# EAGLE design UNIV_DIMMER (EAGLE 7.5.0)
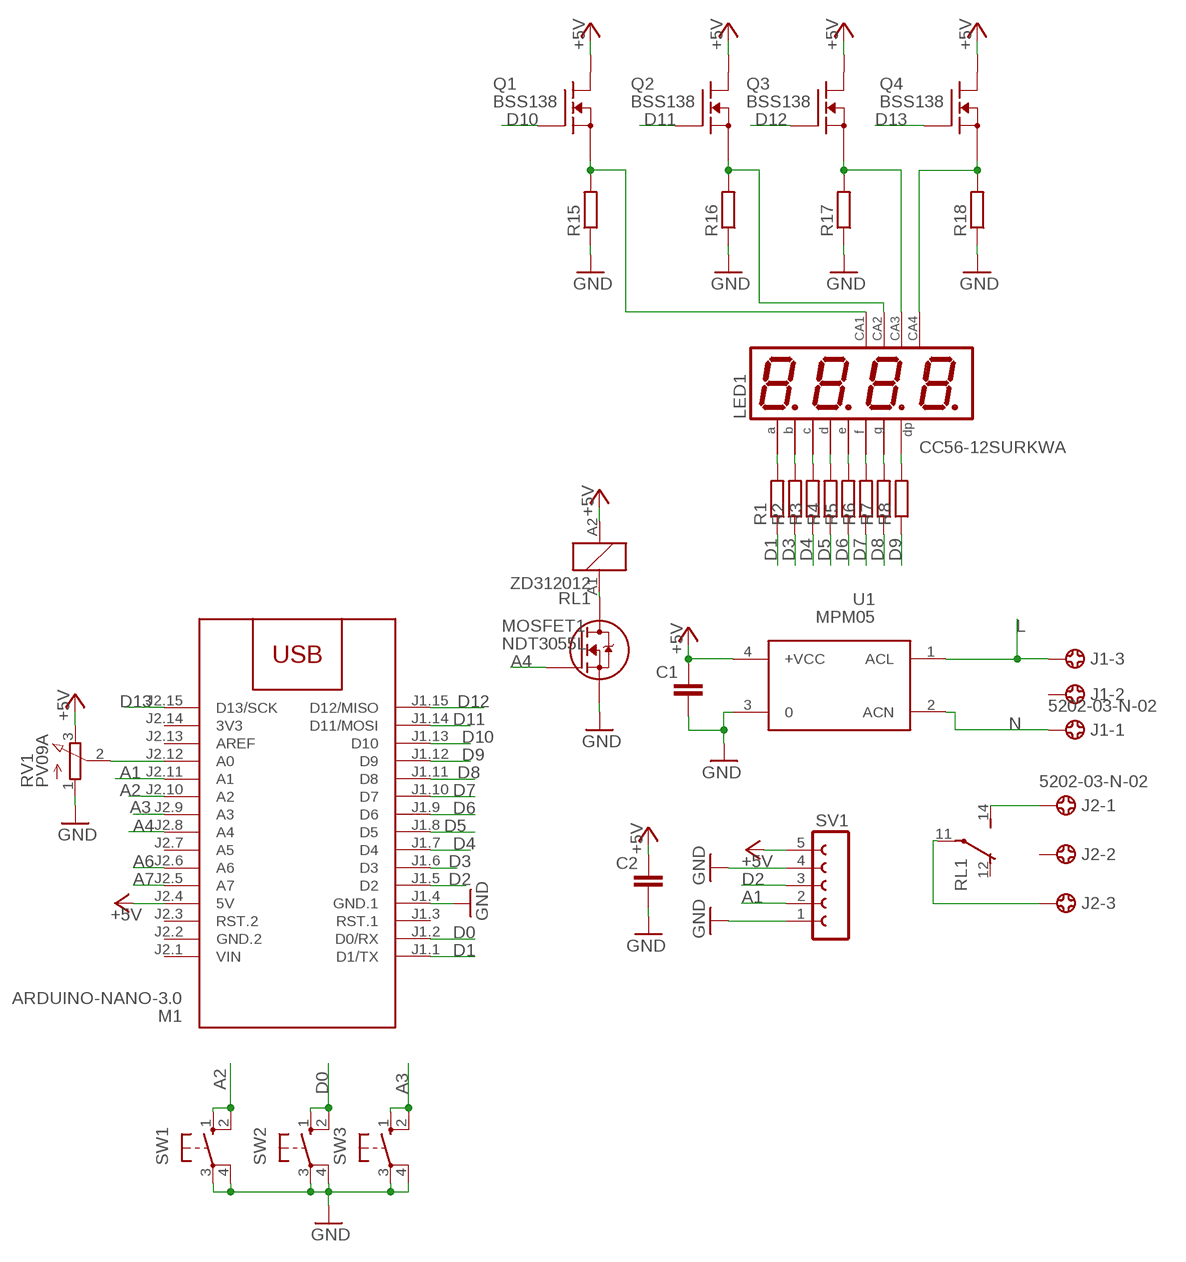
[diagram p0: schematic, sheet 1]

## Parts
C1  C-EUC1206  [C1206]
C2  C-EUC1206  [C1206]
J1  5202-03-N-02  [5202-03-N-02]
J2  5202-03-N-02  [5202-03-N-02]
LED1  CC56-12SURKWA  CA56-12SURKWA  [CA56-12SURKWA]
M1  ARDUINO-NANO-3.0  [ARDUINO-NANO-3.0]
MOSFET1  NDT3055L  [SOT223-4]
Q1  BSS138  [SOT23]
Q2  BSS138  [SOT23]
Q3  BSS138  [SOT23]
Q4  BSS138  [SOT23]
R1  R-EU_R1206  [R1206]
R2  R-EU_R1206  [R1206]
R3  R-EU_R1206  [R1206]
R4  R-EU_R1206  [R1206]
R5  R-EU_R1206  [R1206]
R6  R-EU_R1206  [R1206]
R7  R-EU_R1206  [R1206]
R8  R-EU_R1206  [R1206]
R15  R-EU_R1206  [R1206]
R16  R-EU_R1206  [R1206]
R17  R-EU_R1206  [R1206]
R18  R-EU_R1206  [R1206]
RL1  ZD312012  [ZD1]
RV1  PV09A  [PTV09]
SV1  FE05-1  [FE05-1]
SW1  10-XX  [B3F-10XX]
SW2  10-XX  [B3F-10XX]
SW3  10-XX  [B3F-10XX]
U1  MPM05  [MPM05]

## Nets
+5V: C1.1 C2.1 M1.J2.4(5V) Q1.2(D) Q2.2(D) Q3.2(D) Q4.2(D) RL1.A2 RV1.3(E) SV1.5 U1.4(+VCC)
A1: M1.J2.11(A1) SV1.2
A2: M1.J2.10(A2) SW1.1(S) SW1.2(S1)
A3: M1.J2.9(A3) SW3.1(S) SW3.2(S1)
A4: M1.J2.8(A4) MOSFET1.1(G)
A6: M1.J2.6(A6)
A7: M1.J2.5(A7)
D0: M1.J1.2(D0/RX) SW2.1(S) SW2.2(S1)
D1: M1.J1.1(D1/TX) R1.1
D2: M1.J1.5(D2) SV1.3
D3: M1.J1.6(D3) R2.1
D4: M1.J1.7(D4) R3.1
D5: M1.J1.8(D5) R4.1
D6: M1.J1.9(D6) R5.1
D7: M1.J1.10(D7) R6.1
D8: M1.J1.11(D8) R7.1
D9: M1.J1.12(D9) R8.1
D10: M1.J1.13(D10) Q1.3(G)
D11: M1.J1.14(D11/MOSI) Q2.3(G)
D12: M1.J1.15(D12/MISO) Q3.3(G)
D13: M1.J2.15(D13/SCK) Q4.3(G)
GND: C1.2 C2.2 M1.J1.4(GND.1) MOSFET1.3(S) R15.1 R16.1 R17.1 R18.1 RV1.1(A) SV1.1 SV1.4 SW1.3(P) SW1.4(P1) SW2.3(P) SW2.4(P1) SW3.3(P) SW3.4(P1) U1.3
L: J1.3 U1.1(ACL)
N: J1.1 U1.2(ACN)
N$1: M1.J2.12(A0) RV1.2(S)
N$2: J2.1 RL1.14(2:S)
N$3: J2.3 RL1.11(2:P)
N$10: LED1.11(A) R1.2
N$11: LED1.7(B) R2.2
N$12: MOSFET1.2(D) MOSFET1.4(D) RL1.A1
N$15: LED1.4(C) R3.2
N$16: LED1.2(D) R4.2
N$17: LED1.1(E) R5.2
N$18: LED1.10(F) R6.2
N$19: LED1.5(G) R7.2
N$20: LED1.3(DP) R8.2
N$21: LED1.12(CA) Q1.1(S) R15.2
N$22: LED1.9(CA) Q2.1(S) R16.2
N$23: LED1.8(CA) Q3.1(S) R17.2
N$24: LED1.6(CA4) Q4.1(S) R18.2
Unconnected: J1.2 J2.2 M1.J1.3(RST.1) M1.J2.3(RST.2) M1.J2.7(A5) M1.J2.13(AREF) RL1.12(2:O)

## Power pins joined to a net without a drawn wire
3V3: M1.J2.14(3V3)
GND.2: M1.J2.2(GND.2)
VIN: M1.J2.1(VIN)

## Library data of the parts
C1 C2 = rcl:C-EU: CAPACITOR, European symbol
J1 J2 = con-ebyelectro:5202-03-N-02: Barrier Blocks Sreies 5202 Source: http://www.ebyelectro.com/PDF/5202-XX-N-02.pdf; OC_FARNELL: unknown; OC_NEWARK: unknown
LED1 = display-kingbright:CA56-12SURKWA
M1 = diy-modules:ARDUINO-NANO-3.0: Arduino Nano 3.0 and compatible devices More details available here: https://www.arduino.cc/en/Main/ArduinoBoardNano Click here to find device on ebay.com
MOSFET1 = NDT3055L:NDT3055L: Trans MOSFET N-CH 60V 4A 4-Pin(3+Tab) SOT-223 Trans MOSFET N-CH 60V 4A 4-Pin(3+Tab) SOT-223 Check availability; AVAILABILITY: In Stock; CHECK_PRICES: https://www.snapeda.com/parts/NDT3055L/Onsemi/view-part/?ref=eda; DESCRIPTION: Trans MOSFET N-CH 60V 4A 4-Pin(3+Tab) SOT-223 Trans MOSFET N-CH 60V 4A 4-Pin(3+Tab) SOT-223; MF: ON; MP: NDT3055L; PACKAGE: SOT-223-4 Fairchild Semiconductor; PRICE: None; SNAPEDA_LINK: https://www.snapeda.com/parts/NDT3055L/Onsemi/view-part/?ref=snap
Q1-Q4 = transistor-fet:BSS138
R1-R8 R15-R18 = rcl:R-EU_: RESISTOR, European symbol
RL1 = relay:ZD?1*: Power Relay SCHRACK 1 pole 30 A Source: http://www.schrack.com/.. 5848.pdf; OC_FARNELL: unknown; OC_NEWARK: unknown
RV1 = pot:PV09A
SV1 = con-lsta:FE05-1: FEMALE HEADER; OC_FARNELL: unknown; OC_NEWARK: unknown
SW1-SW3 = switch-omron:10-XX: OMRON SWITCH; MPN: B3F-1000; OC_FARNELL: 176432; OC_NEWARK: 36M3542
U1 = acdc:MPM05: AC DC Converter 5W

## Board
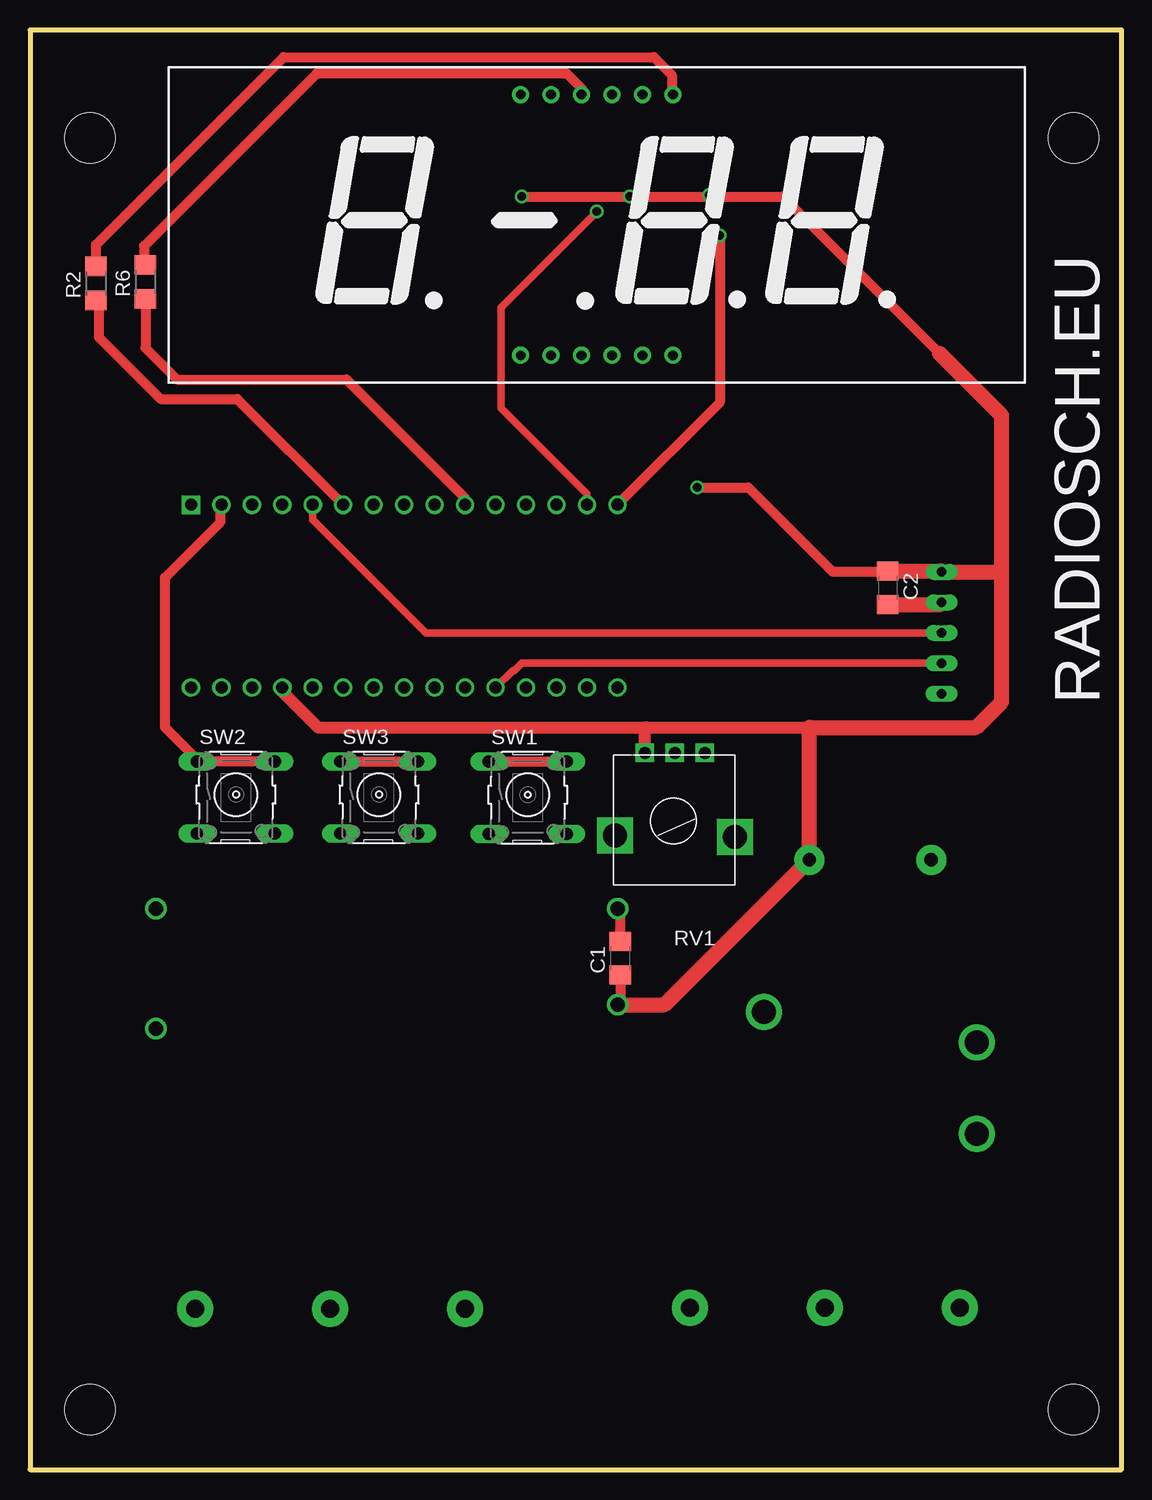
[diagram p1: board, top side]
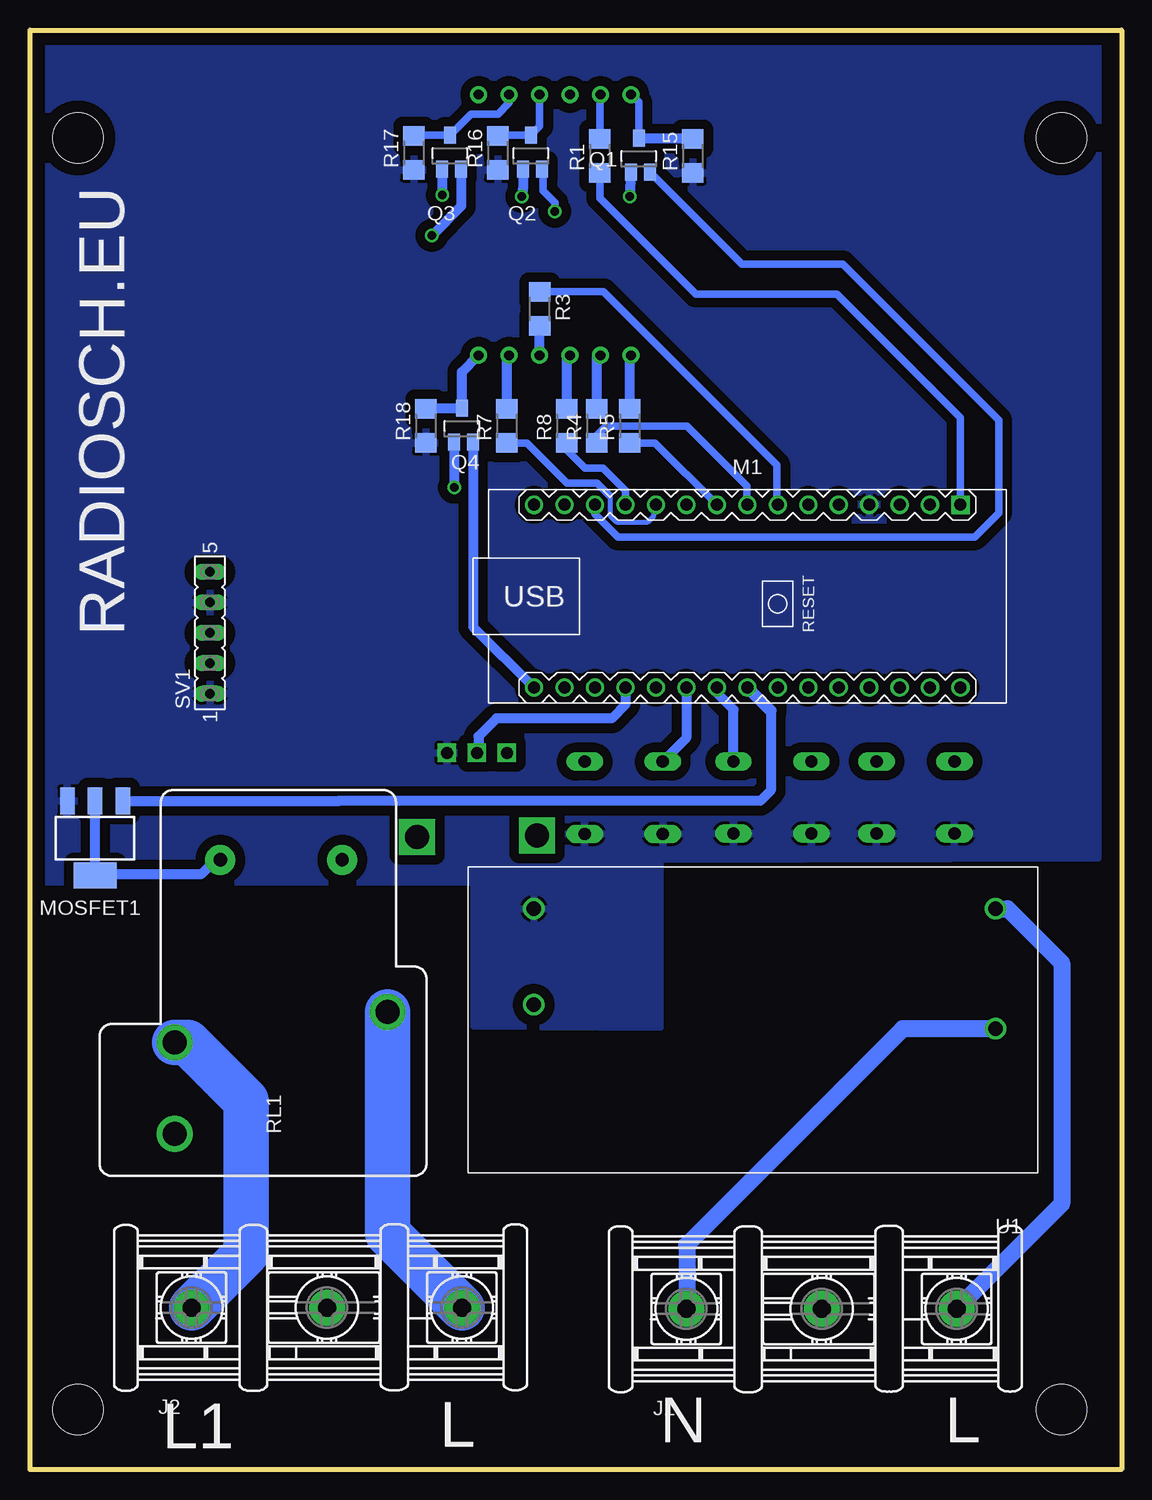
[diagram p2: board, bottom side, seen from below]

Size 91 x 120 mm. Coordinates in mm from the lower left corner, seen from the top.
Outline: 0,0 91,0 91,120 0,120 0,0
Copper layers (1*16): Top 0.035mm / dielectric 1.5mm / Bottom 0.035mm
Design rules "default": minimum track width 10mil, minimum drill 24mil, track to track 8mil, track to pad 8mil, pad to pad 8mil, via to via 8mil, smd to smd 8mil, copper to edge 40mil, drill to drill 8mil, minimum pad ring 10mil, minimum via ring 8mil, stop-mask expansion 4mil, vias tented up to drill 0mil, thermal gap 10mil
Holes 4.2 mm at 5,111 5,5 87,111 87,5

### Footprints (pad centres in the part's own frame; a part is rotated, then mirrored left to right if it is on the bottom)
C1206 = smd 1.6 x 1.8: 1 -1.4,0; 2 1.4,0
5202-03-N-02 = drill 1.5 pad 3: 1 -9.29,0; 2 2,0; 3 13.25,0
CA56-12SURKWA = drill 0.8 pad 1.422: 1 10.65,-7.12; 2 13.19,-7.12; 3 15.73,-7.12; 4 18.27,-7.12; 5 20.81,-7.12; 6 23.35,-7.12; 7 23.35,14.62; 8 20.81,14.62; 9 18.27,14.62; 10 15.73,14.62; 11 13.19,14.62; 12 10.65,14.62
ARDUINO-NANO-3.0 = drill 1 square: J1.1 17.78,7.62 | drill 1: J1.2 15.24,7.62; J1.3 12.7,7.62; J1.4 10.16,7.62; J1.5 7.62,7.62; J1.6 5.08,7.62; J1.7 2.54,7.62; J1.8 0,7.62; J1.9 -2.54,7.62; J1.10 -5.08,7.62; J1.11 -7.62,7.62; J1.12 -10.16,7.62; J1.13 -12.7,7.62; J1.14 -15.24,7.62; J1.15 -17.78,7.62; J2.1 17.78,-7.62; J2.2 15.24,-7.62; J2.3 12.7,-7.62; J2.4 10.16,-7.62; J2.5 7.62,-7.62; J2.6 5.08,-7.62; J2.7 2.54,-7.62; J2.8 0,-7.62; J2.9 -2.54,-7.62; J2.10 -5.08,-7.62; J2.11 -7.62,-7.62; J2.12 -10.16,-7.62; J2.13 -12.7,-7.62; J2.14 -15.24,-7.62; J2.15 -17.78,-7.62
SOT223-4 = smd 1.219 x 2.235: 1 -2.24,-3.091; 2 0.071,-3.091; 3 2.383,-3.091 | smd 3.6 x 2.2: 4 0.071,3.107
SOT23 = smd 1 x 1.4: 1 0,1.735; 2 -0.632,-1.1; 3 0.95,-1.1
R1206 = smd 1.6 x 1.803: 1 -1.422,0; 2 1.422,0
ZD1 = drill 2 pad 2.5: 11 -2.54,-8.88; 12 -12.7,8.88; 14 -5.08,8.88 | drill 1.1 pad 2.5: A1 10.16,5.08; A2 10.16,-5.08
PTV09 = drill 1 square: 1 -2.5,0; 2 0,0; 3 2.5,0 | drill 2 square: P$4 -5,7; P$5 5,6.9
FE05-1 = drill 0.813 long: 1 -5.08,0; 2 -2.54,0; 3 0,0; 4 2.54,0; 5 5.08,0
B3F-10XX = drill 1.016 long: 1 -3.251,2.761; 2 3.251,2.761; 3 -3.251,-3.261; 4 3.251,-3.261
MPM05 = drill 1.2: 1 3.5,-22; 2 3.5,-12; 3 42,-22; 4 42,-14

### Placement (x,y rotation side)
C1  49.22,42.62 90 top
C2  71.5,73.5 270 top
J1  27,13.39 0 bottom
J2  68.25,13.5 0 bottom
LED1  30.25,100 0 top
M1  31.2,72.8 0 bottom
MOSFET1  85.5,52.62 180 bottom
Q1  40.25,109.25 0 bottom
Q2  49.25,109.5 0 bottom
Q3  56,109.5 0 bottom
Q4  55,86.75 0 bottom
R1  43.5,109.5 90 bottom
R2  5.5,98.88 90 top
R3  48.5,96.75 270 bottom
R4  43.75,87 90 bottom
R5  41,87 90 bottom
R6  9.62,99 90 top
R7  51.25,87 90 bottom
R8  46.25,87 90 bottom
R15  35.75,109.5 90 bottom
R16  52,109.75 90 bottom
R17  59,109.75 90 bottom
R18  58,87 90 bottom
RL1  70.05,40.67 90 bottom
RV1  53.75,59.75 180 top
SV1  76,69.75 90 bottom
SW1  41.5,56.25 0 top
SW2  17.17,56.27 0 top
SW3  29.1,56.27 0 top
U1  7,24.75 180 bottom

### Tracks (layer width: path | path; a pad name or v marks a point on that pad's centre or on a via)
+5V  (via drill 0.7)
  Top 0.813: v41,106.12 v50,106.12 56.5,106.12 | 56.5,106.12 v56.62,106.25 | 56.5,106.12 62.75,106.12 75.81,93.06 76,92.88 | v55.62,81.88 59.88,81.88 66.88,74.88 71.47,74.88 C2.1 | C1.1 49.22,38.97 U1.4
  Top 1.016: M1.J2.4 21.04,64.84 24,61.88 51.38,61.88 | 51.38,61.88 65,61.88 | RV1.3 51.25,61.75 51.38,61.88
  Top 1.27: U1.4 52.89,38.75 RL1.A2 64.97,61.84 65,61.88 78.88,61.88 81,64 81,74.75 | 81,74.75 81,87.88 75.81,93.06 | 81,74.75 80.92,74.83 SV1.5 75.93,74.9 C2.1
  Bottom 0.61: 55.5,81.75 v55.62,81.88
  Bottom 0.813: v41,106.12 Q1.2 | Q2.2 49.88,107.01 v50,106.12 | Q3.2 56.63,107.12 v56.62,106.25 | Q4.2 55.63,81.88 v55.62,81.88
A1
  Top 0.61: M1.J2.11 40.27,66.62 40.38,66.62 41,67.25 75.96,67.25 SV1.2
A2
  Top 0.813: SW1.1 SW1.2
  Bottom 0.813: M1.J2.10 36.28,60.98 SW1.1
A3
  Top 0.813: SW3.1 SW3.2
  Bottom 0.813: SW3.2 32.35,63.35 33.62,64.62 33.62,65.06 M1.J2.9
A4
  Bottom 0.813: 29.25,63.23 29.25,56.62 30.12,55.75 65.25,55.75 65.28,55.72 MOSFET1.1
  Bottom 1.016: 29.25,63.23 M1.J2.8
D0
  Top 0.813: M1.J1.2 15.88,80.33 15.88,79 11.25,74.38 11.25,61.88 13.92,59.21 SW2.1 SW2.2
D1
  Bottom 0.61: M1.J1.1 13.42,87.67 23.75,98 35.5,98 43.5,106 R1.1
D2
  Top 0.61: M1.J1.5 23.58,79.17 33,69.75 SV1.3
D3
  Top 0.813: R2.1 5.75,97.2 5.75,94.38 10.88,89.25 17.29,89.25 M1.J1.6
D4
  Bottom 0.61: R3.1 43.17,98.17 28.75,83.75 28.75,80.51 M1.J1.7
D5
  Bottom 0.61: M1.J1.8 31.25,80.47 31.25,82 36.25,87 43,87 43.75,86.25 R4.1
D6
  Bottom 0.61: R5.1 38.9,85.58 M1.J1.9
D7
  Top 0.813: R6.1 9.62,93.5 12.25,90.88 26.38,90.88 36.25,81 36.25,80.45 M1.J1.10
D8
  Bottom 0.406: M1.J1.11 39,80.24 39,79.5 39.5,79 42.12,79 42.62,79.5 42.62,81.12 42.75,81.25
  Bottom 0.61: R7.1 49.58,85.58 46.25,82.25 43.75,82.25 42.75,81.25
D9
  Bottom 0.61: M1.J1.12 41.36,81.61 43.25,83.5 44.75,83.5 46.25,85 R8.1
D10
  Bottom 0.61: M1.J1.13 43.9,79.65 42,77.75 12.25,77.75 10.25,79.75 10.25,87.5 23.25,100.5 31.65,100.5 Q1.3
D11  (via drill 0.7)
  Top 0.61: M1.J1.14 46.44,81.31 39.25,88.5 39.25,96.88 v47.25,104.88
  Bottom 0.61: v47.25,104.88 47.25,105.62 48.25,106.62 48.25,108.35 Q2.3
D12  (via drill 0.7)
  Top 0.813: v57.5,102.88 57.5,88.94 M1.J1.15
  Bottom 0.813: Q3.3 55.05,105.33 v57.5,102.88
D13
  Bottom 0.813: Q4.3 54.05,70.25 M1.J2.15
GND
  Top 0.813: C1.2 49.22,46.53 U1.3
  Top 1.27: C2.2 75.81,72.1 SV1.4
  pour Bottom (isolate 0.813): 2,119 90,119 90,49 54,49 54,37 38.5,36.88 38.5,50.88 2,51
L
  Bottom 1.422: U1.1 9.5,46.75 5,42.25 5,22.14 J1.3
N
  Bottom 1.422: U1.2 18.25,36.75 36.25,18.75 36.25,13.43 J1.1
N$1
  Bottom 0.813: M1.J2.12 41.36,63.77 42.5,62.62 52.12,62.62 53.62,61.12 53.62,59.88 RV1.2
N$2
  Bottom 3.81: RL1.14 77.84,35.59 73,30.75 73,18.04 J2.1
N$3
  Bottom 3.81: RL1.11 61.17,19.67 J2.3
N$10
  Bottom 0.61: R1.2 43.5,114.56 LED1.11
N$11
  Top 0.813: R2.2 5.5,102.12 21.12,117.75 52,117.75 53.5,116.25 53.5,114.72 LED1.7
N$12
  Bottom 0.813: MOSFET1.2 MOSFET1.4 85.47,49.62 76.75,49.62 75.55,50.83 RL1.A1
N$15
  Bottom 0.813: LED1.4 48.52,95.31 R3.2
N$16
  Bottom 0.813: R4.2 43.75,92.57 LED1.2
N$17
  Bottom 0.813: R5.2 41,92.78 LED1.1
N$18
  Top 0.813: LED1.10 45.98,115.14 44.75,116.38 23.88,116.38 9.5,102 9.5,100.55 R6.2
N$19
  Bottom 0.813: R7.2 51.25,92.69 LED1.5
N$20
  Bottom 0.813: R8.2 46.25,92.61 LED1.3
N$21
  Bottom 0.61: Q1.1 40.25,113.97 LED1.12
  Bottom 0.813: R15.2 40.19,110.92 Q1.1
N$22
  Bottom 0.61: LED1.9 48.52,111.97 Q2.1 51.94,111.23 R16.2
N$23
  Bottom 0.61: LED1.8 51.06,113.94 52,113 54.23,113 Q3.1 58.94,111.23 R17.2
N$24
  Bottom 0.61: 55.06,88.42 Q4.1
  Bottom 0.813: 55.06,88.42 R18.2 | Q4.1 55,91.48 LED1.6

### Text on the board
tPlace: RADIOSCH.EU
bPlace: RADIOSCH.EU | L | N | L | L1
